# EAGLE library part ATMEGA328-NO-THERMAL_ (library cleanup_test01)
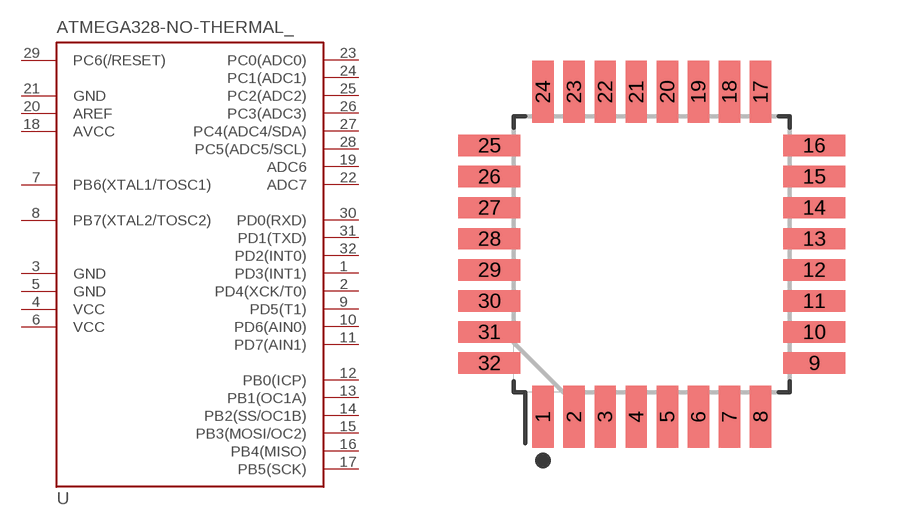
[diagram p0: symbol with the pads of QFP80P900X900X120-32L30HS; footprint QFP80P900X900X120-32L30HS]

Designator prefix -

## ATMEGA328-NO-THERMAL_32TQFP  [QFP80P900X900X120-32L30HS]
1  PD3(INT1)
2  PD4(XCK/T0)
3  GND  pwr
4  VCC  pwr
5  GND  pwr
6  VCC  pwr
7  PB6(XTAL1/TOSC1)
8  PB7(XTAL2/TOSC2)
9  PD5(T1)
10  PD6(AIN0)
11  PD7(AIN1)
12  PB0(ICP)
13  PB1(OC1A)
14  PB2(SS/OC1B)
15  PB3(MOSI/OC2)
16  PB4(MISO)
17  PB5(SCK)
18  AVCC  pwr
19  ADC6
20  AREF  pas
21  GND  pwr
22  ADC7
23  PC0(ADC0)
24  PC1(ADC1)
25  PC2(ADC2)
26  PC3(ADC3)
27  PC4(ADC4/SDA)
28  PC5(ADC5/SCL)
29  PC6(/RESET)
30  PD0(RXD)
31  PD1(TXD)
32  PD2(INT0)

## Footprint QFP80P900X900X120-32L30HS (pad centres in mm)
smd 0.55 x 1.6: 1 -2.8,-4.18; 2 -2,-4.18; 3 -1.2,-4.18; 4 -0.4,-4.18; 5 0.4,-4.18; 6 1.2,-4.18; 7 2,-4.18; 8 2.8,-4.18; 17 2.8,4.18; 18 2,4.18; 19 1.2,4.18; 20 0.4,4.18; 21 -0.4,4.18; 22 -1.2,4.18; 23 -2,4.18; 24 -2.8,4.18
smd 1.6 x 0.55: 9 4.18,-2.8; 10 4.18,-2; 11 4.18,-1.2; 12 4.18,-0.4; 13 4.18,0.4; 14 4.18,1.2; 15 4.18,2; 16 4.18,2.8; 25 -4.18,2.8; 26 -4.18,2; 27 -4.18,1.2; 28 -4.18,0.4; 29 -4.18,-0.4; 30 -4.18,-1.2; 31 -4.18,-2; 32 -4.18,-2.8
